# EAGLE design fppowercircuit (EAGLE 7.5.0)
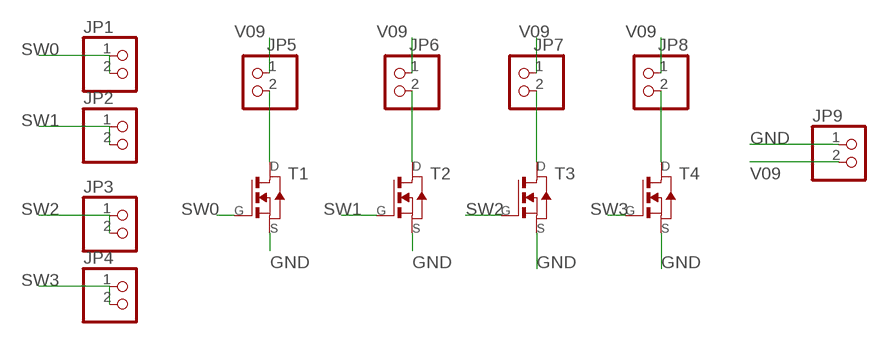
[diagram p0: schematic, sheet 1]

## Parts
JP1  PINHD-1X2  [1X02]
JP2  PINHD-1X2  [1X02]
JP3  PINHD-1X2  [1X02]
JP4  PINHD-1X2  [1X02]
JP5  PINHD-1X2  [1X02]
JP6  PINHD-1X2  [1X02]
JP7  PINHD-1X2  [1X02]
JP8  PINHD-1X2  [1X02]
JP9  PINHD-1X2  [1X02]
T1  NMOSFETSOT23  [SOT-23]
T2  NMOSFETSOT23  [SOT-23]
T3  NMOSFETSOT23  [SOT-23]
T4  NMOSFETSOT23  [SOT-23]

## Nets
GND: JP9.1 T1.2(S) T2.2(S) T3.2(S) T4.2(S)
N$5: JP5.2 T1.1(D)
N$7: JP8.2 T4.1(D)
N$9: JP6.2 T2.1(D)
N$11: JP7.2 T3.1(D)
SW0: JP1.1 JP1.2 T1.3(G)
SW1: JP2.1 JP2.2 T2.3(G)
SW2: JP3.1 JP3.2 T3.3(G)
SW3: JP4.1 JP4.2 T4.3(G)
V09: JP5.1 JP6.1 JP7.1 JP8.1 JP9.2

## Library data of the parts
JP1-JP9 = pinhead:PINHD-1X2: PIN HEADER
T1-T4 = fab:NMOSFET: MOS FET

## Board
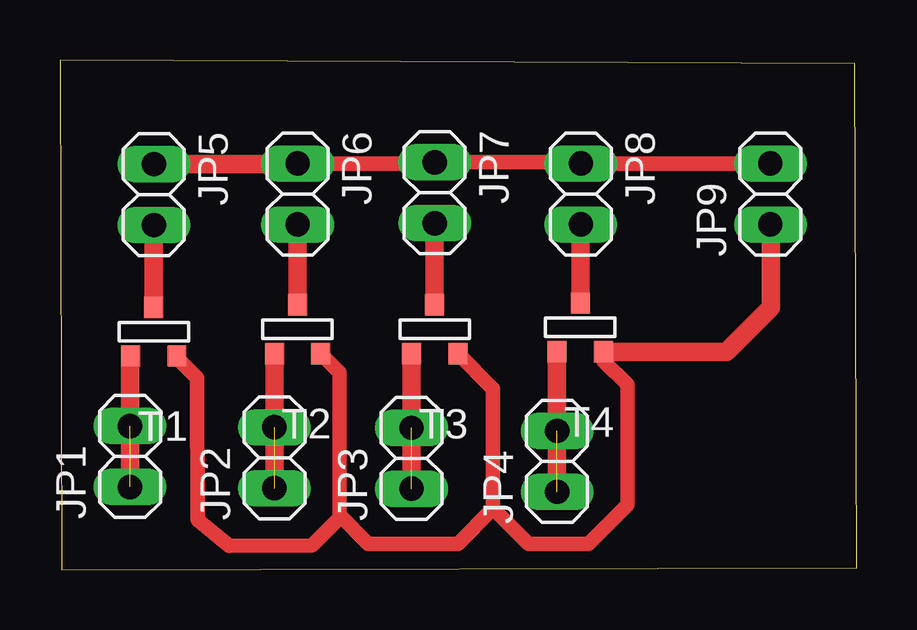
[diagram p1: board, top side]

Size 33.23 x 21.26 mm. Coordinates in mm from the lower left corner, seen from the top.
Outline: 0.08,0 33.23,0.08 33.13,21.11 0,21.26 0.08,0
Copper layers (1*16): Top 0.035mm / dielectric 1.5mm / Bottom 0.035mm
Design rules "default *": minimum track width 10mil, minimum drill 24mil, track to track 12mil, track to pad 12mil, pad to pad 12mil, via to via 12mil, smd to smd 12mil, copper to edge 40mil, drill to drill 8mil, minimum pad ring 10mil, minimum via ring 8mil, stop-mask expansion 4mil, vias tented up to drill 0mil, thermal gap 10mil

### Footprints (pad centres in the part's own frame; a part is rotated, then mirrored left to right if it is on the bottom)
1X02 = drill 1.016 long: 1 -1.27,0; 2 1.27,0
SOT-23 = smd 0.787 x 0.889: 1 0.025,-1.016; 2 -0.94,1.016; 3 0.991,1.016

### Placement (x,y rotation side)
JP1  2.92,4.72 90 top
JP2  8.94,4.67 90 top
JP3  14.66,4.65 90 top
JP4  20.73,4.52 90 top
JP5  3.91,15.65 270 top
JP6  9.91,15.67 270 top
JP7  15.62,15.72 270 top
JP8  21.72,15.67 270 top
JP9  29.62,15.67 90 top
T1  3.94,9.93 180 top
T2  9.93,10.03 180 top
T3  15.65,10.03 180 top
T4  21.72,10.11 180 top

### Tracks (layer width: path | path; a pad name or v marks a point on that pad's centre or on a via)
GND
  Top 0.61: 10.85,8.99 T2.2 11.66,8.23 11.66,2.29 | 29.64,14.38 JP9.1 | T4.2 22.66,8.71 23.65,7.72 23.65,2.72 22.02,1.09 19.53,1.09 18.06,2.57 | 18.06,2.57 18.06,7.54 T3.2 | T1.2 4.88,8.84 5.72,8 5.74,2.08 7.06,0.99 10.52,1.02 11.66,2.16 11.66,2.29 | 11.66,2.29 12.85,1.09 16.59,1.09 18.06,2.57
  Top 0.762: T4.2 27.79,9.09 29.64,10.95 29.64,14.38
N$5
  Top 0.762: T1.1 JP5.2
N$7
  Top 0.61: JP8.2 21.69,14.4
  Top 0.762: 21.69,14.4 T4.1
N$9
  Top 0.762: T2.1 JP6.2
N$11
  Top 0.762: JP7.2 T3.1
SW0  (1 unrouted)
  Top 0.61: T1.3 2.92,8.92
  Top 0.762: 2.92,8.92 JP1.1
SW1  (1 unrouted)
  Top 0.762: JP2.1 T2.3
SW2  (1 unrouted)
  Top 0.762: JP3.1 T3.3
SW3  (1 unrouted)
  Top 0.762: JP4.1 T4.3
V09
  Top 0.61: 9.91,16.92 JP6.1 15.62,16.94 JP7.1 21.72,16.99 JP8.1 JP9.2
  Top 0.762: JP5.1 9.91,16.92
